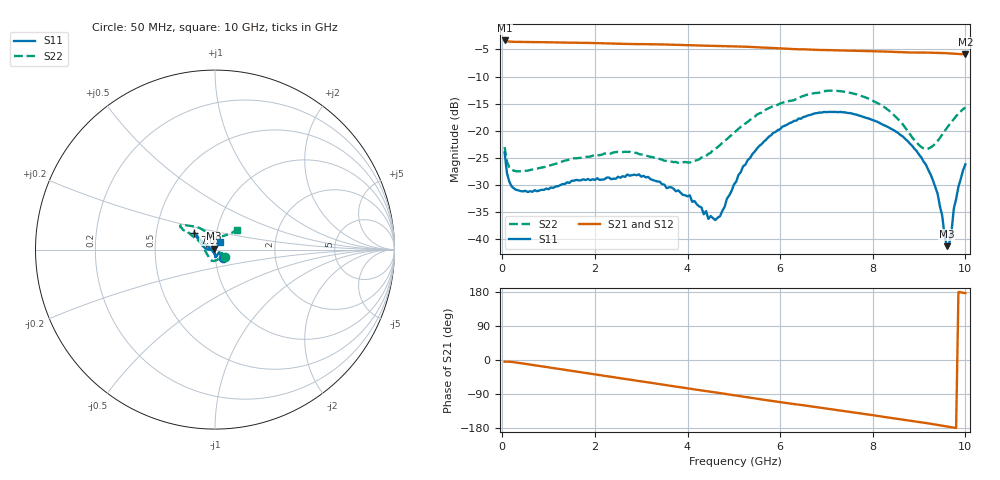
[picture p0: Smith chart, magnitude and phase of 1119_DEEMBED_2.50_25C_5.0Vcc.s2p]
!Hittite Microwave Corp.
!Digital Attenuator/PhaseShifter Rev 1.4.0
!Filename: C:\DATA\DATA\1119_DEEMBED_2.50_25C_5.0Vcc.s2p
!VNA ID: Agilent Technologies,N5224A,MY51441122,A.10.45.03
!Device type:
!2 Port Calibration.
!Temp(C): 25
!Lot Number:
!Serial Number:
!Operator:
!Misc:
!Attenuator:  2.500
# GHZ S DB R 50.0
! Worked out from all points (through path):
!   200 points, 50 MHz to 10 GHz, reference 50 ohm
!   highest |S21| = -3.35 dB at 50 MHz (marker M1); lowest = -5.9 dB at 10 GHz (marker M2)
!   group delay of S21, straight-line fit = 50.1 ps
!   lowest |S11| = -41.2 dB at 9.6 GHz (marker M3), VSWR 1.02, Z = 49.3 + j0.548 ohm
!   |S11| at or under -10 dB: start of sweep to end of sweep
!   |S22| runs from -27.5 to -12.6 dB; largest |S21 - S12| = 0.0022
!   S11 on the Smith chart (normalised r, x): 50 MHz: 1.08, -0.10; 7.05 GHz: 0.78, +0.15; 10 GHz: 1.05, +0.09
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0.05  -23.94 -48.0  -3.35 -4.6  -3.35 -4.6  -22.98 -37.0
0.1  -27.74 -42.7  -3.52 -4.1  -3.52 -4.1  -25.64 -31.3
0.15  -29.32 -37.6  -3.56 -4.5  -3.56 -4.5  -26.67 -27.3
0.3  -30.87 -31.1  -3.61 -6.7  -3.61 -6.7  -27.43 -25.3
1.75  -28.91 -78.9  -3.79 -33.5  -3.78 -33.5  -24.84 -73.5
2.95  -28.00 -87.6  -4.01 -55.4  -4.02 -55.4  -24.27 -115.1
3.4  -29.35 -90.1  -4.07 -63.7  -4.08 -63.8  -25.18 -129.9
4.05  -31.86 -92.2  -4.22 -75.6  -4.23 -75.7  -25.83 -160.0
4.6  -36.42 -141.6  -4.36 -85.6  -4.38 -85.7  -23.32 165.9
5.05  -29.36 162.5  -4.45 -93.8  -4.47 -93.8  -20.01 152.1
5.2  -26.54 155.6  -4.49 -96.6  -4.51 -96.6  -18.94 150.1
5.75  -21.10 147.9  -4.69 -106.7  -4.71 -106.8  -15.83 148.1
6.7  -16.91 141.3  -5.04 -122.9  -5.05 -123.0  -13.12 147.2
7.05  -16.51 140.8  -5.13 -128.8  -5.14 -128.8  -12.60 145.7
8.35  -19.39 149.5  -5.42 -152.0  -5.42 -152.0  -16.26 127.0
9.15  -26.27 175.9  -5.59 -166.3  -5.60 -166.3  -23.34 92.0
9.400001  -31.58 -179.0  -5.62 -171.2  -5.64 -171.3  -21.86 65.2
9.6  -41.23 140.3  -5.71 -175.4  -5.72 -175.4  -19.46 50.7
9.65  -40.83 95.7  -5.73 -176.4  -5.74 -176.4  -18.90 48.3
9.75  -34.32 63.0  -5.78 -178.5  -5.79 -178.5  -17.82 45.4
9.85  -30.27 58.3  -5.83 179.5  -5.84 179.5  -16.81 43.7
10  -26.16 56.7  -5.92 176.4  -5.93 176.5  -15.69 42.0
